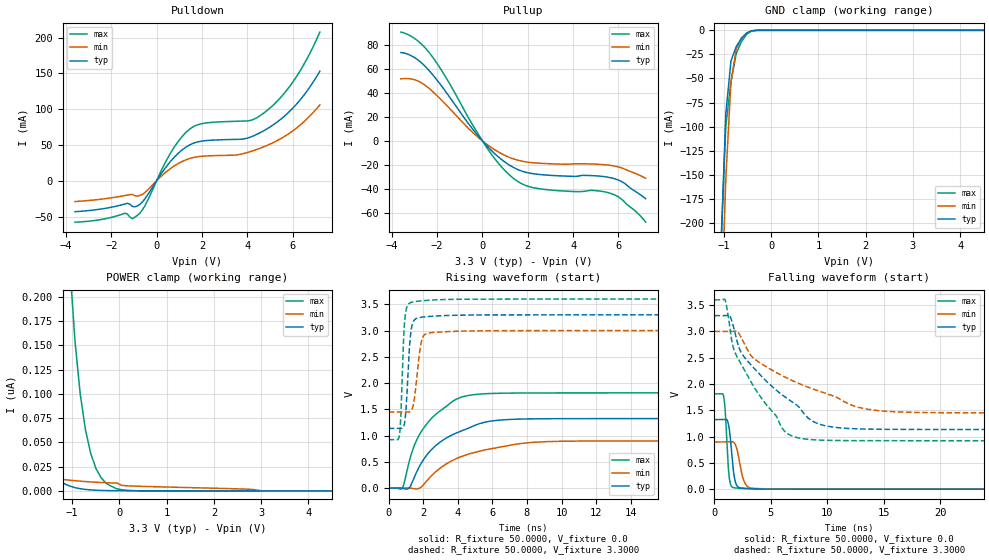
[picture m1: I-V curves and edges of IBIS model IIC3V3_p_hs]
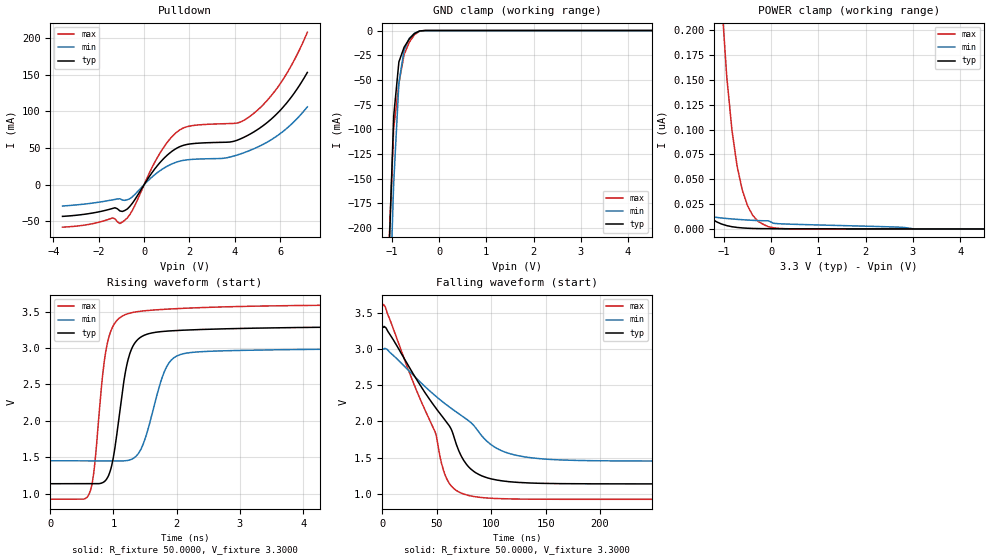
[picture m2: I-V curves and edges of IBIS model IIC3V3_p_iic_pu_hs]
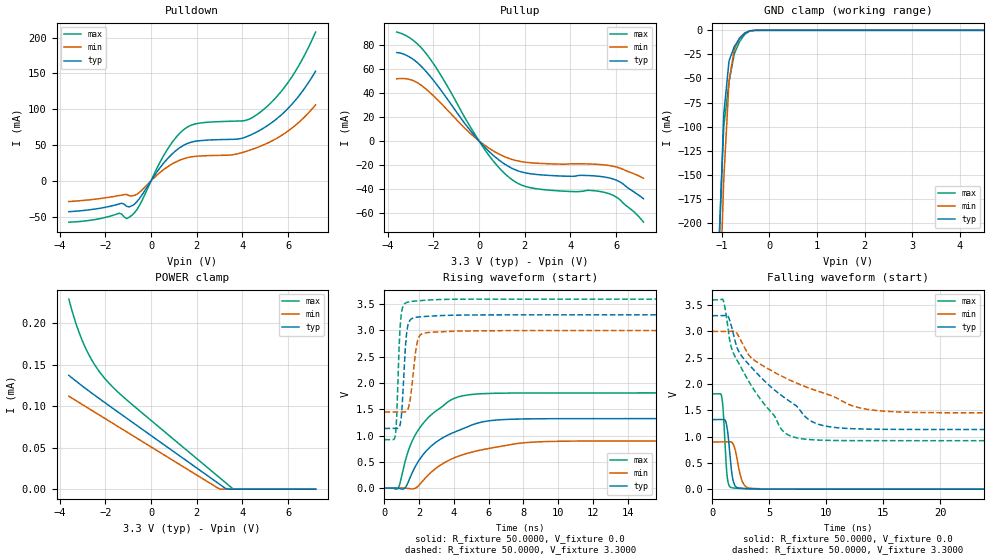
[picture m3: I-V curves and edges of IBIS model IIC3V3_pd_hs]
| IBIS file qfn48_3p3v.ibs generated by Viper version: 2020.12.17
[IBIS Ver]   5.0
[Comment Char]   |_char
[File Name]   qfn48_3p3v.ibs
[File Rev]   1.3
[Date]   Thu Dec 17 17:48:23 2020
[Source]   NXP Viper 2020.12.17
[Notes]
[Disclaimer] IMPORTANT NOTICE
  This information is provided on an AS IS basis and without warranty.
  IN NO EVENT SHALL NXP BE LIABLE FOR INCIDENTAL OR CONSEQUENTIAL
  DAMAGES ARISING FROM USE OF THIS INFORMATION. THIS DISCLAIMER OF
  WARRANTY EXTENDS TO THE USER OF THE INFORMATION, AND TO THEIR CUSTOMERS
  OR USERS OF PRODUCTS  AND IS IN LIEU OF ALL WARRANTIES WHETHER EXPRESS,
  IMPLIED, OR STATUTORY, INCLUDING IMPLIED WARRANTIES OF MERCHANTABILITY
  OR FITNESS FOR PARTICULAR PURPOSE.
  NXP does not represent or warrant that the information furnished
  hereunder is free of infringement of any third party patents,
  copyrights, trade secrets, or other intellectual property rights.
  NXP does not represent or warrant that the information is free of
  defect, or that it meets any particular standard, requirements or need
  of the user of the infomation or their customers.
  NXP reserves the right to change the information in this file
  without notice.
   http://www.nxp.com
[Copyright]   (C) Copyright NXP 2004 - 2020, All Rights Reserved.
|   qfn48
[Component]   qfn48
[Manufacturer]   NXP
[Package]
| variable   typ   min   max
R_pkg   0.17546   0.085233   0.21913
L_pkg   1.979e-9   1.305e-9   2.456e-9
C_pkg   2.005e-13   1.705e-13   3.136e-13
[Pin] signal_name   model_name   R_pin   L_pin   C_pin
1   OPAMP2_INN   NC   0.19686   2.31e-9   1.975e-13
2   P0_1   gpio   0.19885   2.125e-9  1.995e-13
3   P1_0   gpio   0.18462   1.924e-9  1.916e-13
4   P0_11   gpio   0.16868   1.868e-9  1.705e-13
5   VDDIO_1   POWER   NA   NA   NA
6   VDDA   POWER   NA   NA   NA
7   VREF_OUT   NC   0.085233  1.305e-9  2.26e-13
8   VREFP   NC   0.088717  1.309e-9  2.417e-13
9   VREFN   GND   NA   NA   NA
10   P0_16   gpio   0.17435   1.987e-9  1.764e-13
11   P0_10   gpio   0.18496   2.194e-9  1.962e-13
12   P0_15   gpio   0.20527   2.456e-9  2.081e-13
13   P0_8   gpio   0.19119   2.293e-9  1.955e-13
14   OPAMP0_INN   NC   0.1741   2.073e-9  2.101e-13
15   P0_27   gpio   0.16311   1.909e-9  1.814e-13
16   OPAMP1_INN   NC   0.16129   1.801e-9  1.909e-13
17   RESETN   gpio   0.16527   1.717e-9  1.895e-13
18   VDD_CORE   POWER   NA   NA   NA
19   P0_17   gpio   0.16074   1.801e-9  1.861e-13
20   P0_7   gpio   0.1631   1.762e-9  1.925e-13
21   VDDIO_1   POWER   NA   NA   NA
22   VSS_MAIN   GND   NA   NA   NA
23   LX   NC   0.10755   1.361e-9  3.136e-13
24   VDD_MAIN_PWR   NC   NA   NA   NA
25   VBAT   NC   0.21039   2.199e-9  2.126e-13
26   P0_0   gpio   0.19752   2.015e-9  2.122e-13
27   P0_9   gpio   0.17432   1.951e-9  1.886e-13
28   P0_18   gpio   0.16396   1.852e-9  1.719e-13
29   P1_1   gpio   0.1654   1.786e-9  1.75e-13
30   P0_26   gpio   0.16144   1.856e-9  1.764e-13
31   P1_2   gpio   0.16991   1.948e-9  1.848e-13
32   P1_3   gpio   0.18887   2.054e-9  1.928e-13
33   P0_24   gpio   0.17001   1.885e-9  1.791e-13
34   P0_13   iic   0.18016   2.084e-9  1.944e-13
35   P0_14   iic   0.19867   2.298e-9  2.017e-13
36   P0_20   gpio   0.21913   2.324e-9  2.127e-13
37   P0_21   gpio   0.20869   2.216e-9  2.193e-13
38   P0_2   gpio   0.21473   2.265e-9  2.308e-13
39   P0_19   gpio   0.18997   2.14e-9   2.172e-13
40   P0_3   gpio   0.17488   1.926e-9  2.022e-13
41   VDDIO_2   POWER   NA   NA   NA
42   P0_4   gpio   0.16342   1.796e-9  1.814e-13
43   P0_6   gpio   0.16772   1.736e-9  1.992e-13
44   P0_5   gpio   0.16504   1.891e-9  1.879e-13
45   P0_29   gpio   0.16929   1.996e-9  1.98e-13
46   P1_11   gpio   0.18558   2.171e-9  1.964e-13
47   P0_30   gpio   0.20664   2.318e-9  2.205e-13
48   P2_1   gpio   0.1989   2.278e-9  1.972e-13
49   VSS   GND   NA   NA   NA
[Pin Mapping]   pulldown_ref   pullup_ref
1   NC   NC
2   VSS   VDDA
3   VSS   VDDA
4   VSS   VDDA
5   NC   VDDIO_1
6   NC   VDDA
7   NC   NC
8   NC   NC
9   VREFN   NC
10   VSS   VDDA
11   VSS   VDDA
12   VSS   VDDA
13   VSS   VDDA
14   NC   NC
15   VSS   VDDA
16   NC   NC
17   VSS   VDDIO_1
18   NC   VDD_CORE
19   VSS   VDDIO_1
20   VSS   VDDIO_1
21   NC   VDDIO_1
22   VSS_MAIN   NC
23   NC   NC
24   NC   NC
25   NC   NC
26   VSS   VDDIO_2
27   VSS   VDDIO_2
28   VSS   VDDIO_2
29   VSS   VDDIO_2
30   VSS   VDDIO_2
31   VSS   VDDIO_2
32   VSS   VDDIO_2
33   VSS   VDDIO_2
34   VSS   VDDIO_2
35   VSS   VDDIO_2
36   VSS   VDDIO_2
37   VSS   VDDIO_2
38   VSS   VDDIO_2
39   VSS   VDDIO_2
40   VSS   VDDIO_2
41   NC   VDDIO_2
42   VSS   VDDIO_2
43   VSS   VDDIO_2
44   VSS   VDDIO_2
45   VSS   VDDIO_2
46   VSS   VDDIO_2
47   VSS   VDDIO_2
48   VSS   VDDA
49   VSS   NC
|*   Model Selector   *
[Model Selector] gpio
MFIO3V3_pd_hs   EPUN=1 EPD=1 EHS=1
MFIO3V3_pd_ls   EPUN=1 EPD=1 EHS=0
MFIO3V3_pu_hs   EPUN=0 EPD=0 EHS=1
MFIO3V3_pu_ls   EPUN=0 EPD=0 EHS=0
MFIO3V3_p_hs   EPUN=1 EPD=0 EHS=1
MFIO3V3_p_ls   EPUN=1 EPD=0 EHS=0
MFIO3V3_r_hs   EPUN=0 EPD=1 EHS=1
MFIO3V3_r_ls   EPUN=0 EPD=1 EHS=0
[Model Selector] iic
IIC3V3_pd_hs   EGP=1 EPUN=1 EPD=1 EHS=1
IIC3V3_pd_ls   EGP=1 EPUN=1 EPD=1 EHS=0
IIC3V3_p_hs   EGP=1 EPUN=1 EPD=0 EHS=1
IIC3V3_p_ls   EGP=1 EPUN=1 EPD=0 EHS=0
IIC3V3_pu_hs   EGP=1 EPUN=0 EPD=0 EHS=1
IIC3V3_pu_ls   EGP=1 EPUN=0 EPD=0 EHS=0
IIC3V3_r_hs   EGP=1 EPUN=0 EPD=1 EHS=1
IIC3V3_r_ls   EGP=1 EPUN=0 EPD=1 EHS=0
IIC3V3_pd_iic_hs   EGP=0 ECS=0 EPUN=1 EPD=1
IIC3V3_p_iic_hs   EGP=0 ECS=0 EPUN=1 EPD=0
IIC3V3_pu_iic_hs   EGP=0 ECS=0 EPUN=0 EPD=0
IIC3V3_r_iic_hs   EGP=0 ECS=0 EPUN=0 EPD=1
IIC3V3_pd_iic_pu_hs   EGP=0 ECS=1 EPUN=1 EPD=1 SSEL=1
IIC3V3_p_iic_pu_hs   EGP=0 ECS=1 EPUN=1 EPD=0 SSEL=1
IIC3V3_pu_iic_pu_hs   EGP=0 ECS=1 EPUN=0 EPD=0 SSEL=1
IIC3V3_r_iic_pu_hs   EGP=0 ECS=1 EPUN=0 EPD=1 SSEL=1
| End [Component] qfn48
| Models and submodels in the file (24): IIC3V3_p_hs (I/O), IIC3V3_p_iic_hs (I/O_open_drain), IIC3V3_p_iic_pu_hs (I/O_open_drain), IIC3V3_p_ls (I/O), IIC3V3_pd_hs (I/O), IIC3V3_pd_iic_hs (I/O_open_drain), IIC3V3_pd_iic_pu_hs (I/O_open_drain), IIC3V3_pd_ls (I/O), IIC3V3_pu_hs (I/O), IIC3V3_pu_iic_hs (I/O_open_drain), IIC3V3_pu_iic_pu_hs (I/O_open_drain), IIC3V3_pu_ls (I/O), IIC3V3_r_hs (I/O), IIC3V3_r_iic_hs (I/O_open_drain), IIC3V3_r_iic_pu_hs (I/O_open_drain), IIC3V3_r_ls (I/O), MFIO3V3_p_hs (I/O), MFIO3V3_p_ls (I/O), MFIO3V3_pd_hs (I/O), MFIO3V3_pd_ls (I/O), MFIO3V3_pu_hs (I/O), MFIO3V3_pu_ls (I/O), MFIO3V3_r_hs (I/O), MFIO3V3_r_ls (I/O)
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[Model] IIC3V3_p_hs
|   Model IIC3V3_p_hs
| This model was characterised for following simulation conditions:
| External (pad) voltage:
|   - Typ: 3.3V,   - Min: 3.0V,   - Max: 3.6V
| Library cells for typ/min/max conditions are connected as defined below:
|  IO - External Pad
|  A - Core Input
|  EN - Output Buffer Enable
|  BOOST - vdde
|  EGP - vdd
|  EHS - vdd
|  ENZI - vdd
|  EPD - gnd
|  EPUN - vdd
|  ZI - NC
|  ZIF - NC
|  gnd - gnd
|  gnde - gnde
|  vdd - vdd
|  vdde - vdde
| All other pins connected to ground
Model_type I/O
Polarity   Non-Inverting
Enable   Active-Low
Vinl =   0.9900V
Vinh =   2.3100V
Vmeas =  1.6500V
Cref =   0.0F
Rref =   1.0000k
Vref =   0.0V
C_comp   3.6227pF   3.4779pF   3.7656pF
|C_comp_pullup   0.9287pF   0.9115pF   0.9356pF
|C_comp_pulldown   2.3426pF   2.4945pF   2.1982pF
[Model Spec]
| variable   typ   min   max
Vinh   0.9900V   0.9000V   1.0800V
Vinl   2.3100V   2.1000V   2.5200V
Vmeas   1.6500V   1.5000V   1.8000V
[Temperature Range]   25.0000   0.1250k   -40.0000
[Voltage Range]   3.3000V   3.0000V   3.6000V
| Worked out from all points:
|   slope of the pulldown table from 0 to 0.495 V, typ, clamps not added: 22 ohm
|   slope of the pullup table from 0 to 0.495 V, typ, clamps not added: 50.2 ohm
|   GND clamp passes 1 mA (typ) near -0.43 V on its own axis
|   rising waveform, R_fixture 50.0000, V_fixture 0.0: 20-80 % time 2.42ns typ, 3.15ns min, 1.81ns max; typ from 0 V to 1.32 V
|   rising waveform, R_fixture 50.0000, V_fixture 3.3000: 20-80 % time 230ps typ, 322ps min, 186ps max; typ from 1.14 V to 3.3 V
|   falling waveform, R_fixture 50.0000, V_fixture 0.0: 20-80 % time 371ps typ, 535ps min, 282ps max; typ from 1.32 V to 0 V
|   falling waveform, R_fixture 50.0000, V_fixture 3.3000: 20-80 % time 5.52ns typ, 7.85ns min, 3.84ns max; typ from 3.3 V to 1.14 V
[Pulldown]
|Voltage   I(typ)   I(min)   I(max)
-3.6V     -43.22mA   -29.09mA   -57.9mA
-1.29V    -31.46mA   -20.15mA   -46.47mA
-1.07V    -35.79mA   -19.19mA   -52.9mA
-850mV    -35.14mA   -21.36mA   -48.43mA
-520mV    -25.35mA   -16.52mA   -35.11mA
580mV     25.81mA    16.3mA     36.8mA
1.24V     45.79mA    28.53mA    65.82mA
1.9V      54.89mA    33.9mA     79.08mA
4.1V      60.56mA    40.39mA    84.05mA
4.76V     70.46mA    47.89mA    95.34mA
6.08V     103.9mA    71.43mA    141.2mA
7.2V      153mA      106.1mA    207.7mA
[Pullup]
|Voltage   I(typ)   I(min)   I(max)
-3.6V     73.7mA     51.87mA    90.79mA
-2.92V    68.56mA    50.58mA    84.45mA
-2.26V    56.64mA    42.24mA    71.49mA
-1.6V     40.55mA    30.05mA    52.55mA
160mV     -3.402mA   -2.371mA   -4.704mA
820mV     -15.2mA    -10.46mA   -21.22mA
1.37V     -22.16mA   -15.02mA   -31.28mA
1.81V     -25.65mA   -17.18mA   -36.45mA
2.47V     -27.92mA   -18.56mA   -39.79mA
5.66V     -30.76mA   -20.47mA   -43.83mA
6.1V      -33.55mA   -22.29mA   -48.04mA
7.2V      -48.27mA   -31.2mA    -67.82mA
[GND_clamp]
|Voltage   I(typ)   I(min)   I(max)
-3.6V     -5.602A    -5.487A    -5.717A
-1.07V    -242mA     -316.8mA   -230.5mA
-960mV    -86.75mA   -154.7mA   -99.48mA
-850mV    -31.81mA   -53.08mA   -53.5mA
-740mV    -16.96mA   -19.87mA   -24.43mA
-630mV    -8.589mA   -7.919mA   -11.88mA
-520mV    -2.996mA   -2.727mA   -4.187mA
-410mV    -432.5uA   -495.8uA   -580.8uA
7.2V      0A         0A         0A
[POWER_clamp]
|Voltage   I(typ)   I(min)   I(max)
-3.6V     2.12uA     118.8nA    63.41uA
-3.03V    844.5nA    61.84nA    27.62uA
-2.37V    225.8nA    29.91nA    8.403uA
-2.04V    102.5nA    21.72nA    4.105uA
-1.82V    57.11nA    17.98nA    2.406uA
-1.49V    21.61nA    14.11nA    975.4nA
-1.05V    4.967nA    11.05nA    231.3nA
-830mV    2.261nA    10.06nA    99.54nA
-720mV    1.525nA    9.658nA    63.01nA
-500mV    718.9pA    8.985nA    23.37nA
-170mV    294.4pA    8.237nA    4.755nA
7.2V      0A         0A         0A
[Ramp]
| variable   typ   min   max
dV/dt_r  0.7941/2.4211n   0.5390/3.1525n   1.0875/1.8120n
dV/dt_f  1.2989/5.5187n   0.9297/7.8507n   1.6070/3.8381n
R_load = 50.0000
[Rising Waveform]
R_fixture= 50.0000
V_fixture= 0.0
V_fixture_min= 0.0
V_fixture_max= 0.0
|time   V(typ)   V(min)   V(max)
0s        2.243nV    52.63nV    27.54nV
783.4ps   -2.546mV   48.23uV    -3.663mV
1.2ns     6.371mV    -1.183mV   516.9mV
1.762ns   400.2mV    -5.572mV   1.005V
2.604ns   772.3mV    274.8mV    1.368V
3.633ns   1.006V     515.9mV    1.636V
5.446ns   1.245V     716.8mV    1.794V
7.589ns   1.314V     845.6mV    1.81V
17.45ns   1.323V     898mV      1.812V
1us       1.323V     898.3mV    1.813V
[Rising Waveform]
R_fixture= 50.0000
V_fixture= 3.3000
V_fixture_min= 3.0000
V_fixture_max= 3.6000
|time   V(typ)   V(min)   V(max)
0s        1.135V     1.45V      921.7mV
627.3ps   1.135V     1.45V      1.012V
700.7ps   1.134V     1.451V     1.326V
903.6ps   1.208V     1.45V      3.068V
1.101ns   2.057V     1.448V     3.484V
1.223ns   2.763V     1.454V     3.525V
1.356ns   3.105V     1.506V     3.542V
2.023ns   3.26V      2.9V       3.57V
4.301ns   3.294V     2.99V      3.597V
1us       3.3V       3V         3.6V
[Falling Waveform]
R_fixture= 50.0000
V_fixture= 0.0
V_fixture_min= 0.0
V_fixture_max= 0.0
|time   V(typ)   V(min)   V(max)
0s        1.323V     898.3mV    1.813V
822ps     1.323V     898.3mV    1.758V
972.4ps   1.326V     898.3mV    1.431V
1.252ns   1.222V     898.1mV    350.6mV
1.476ns   816.9mV    900.3mV    64.93mV
1.726ns   277.3mV    889.4mV    27.64mV
2.019ns   57.27mV    737.3mV    19.74mV
2.754ns   14.85mV    95.71mV    10.98mV
4.273ns   3.379mV    7.479mV    1.748mV
1us       13.95nV    73.04nV    34.74nV
[Falling Waveform]
R_fixture= 50.0000
V_fixture= 3.3000
V_fixture_min= 3.0000
V_fixture_max= 3.6000
|time   V(typ)   V(min)   V(max)
0s        3.3V       3V         3.6V
933.7ps   3.299V     3V         3.603V
1.389ns   3.287V     2.999V     3.037V
1.891ns   2.917V     3.01V      2.567V
2.697ns   2.498V     2.747V     2.246V
6.123ns   1.774V     2.146V     1.125V
10.95ns   1.17V      1.732V     925.1mV
14.46ns   1.14V      1.495V     922mV
24.74ns   1.135V     1.451V     921.7mV
1us       1.135V     1.45V      921.7mV
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[Model] IIC3V3_p_iic_pu_hs
|   Model IIC3V3_p_iic_pu_hs
| This model was characterised for following simulation conditions:
| External (pad) voltage:
|   - Typ: 3.3V,   - Min: 3.0V,   - Max: 3.6V
| Library cells for typ/min/max conditions are connected as defined below:
|  IO - External Pad
|  A - Core Input
|  EN - Output Buffer Enable
|  BOOST - vdde
|  ECS - vdd
|  EGP - gnd
|  ENZI - vdd
|  EPD - gnd
|  EPUN - vdd
|  SSEL - vdd
|  ZI - NC
|  ZIF - NC
|  gnd - gnd
|  gnde - gnde
|  vdd - vdd
|  vdde - vdde
| All other pins connected to ground
Model_type I/O_open_drain
Polarity   Non-Inverting
Enable   Active-Low
Vinl =   0.9900V
Vinh =   2.3100V
Vmeas =  1.6500V
Cref =   0.0F
Rref =   1.0000k
Vref =   3.3000V
C_comp   3.6227pF   3.4779pF   3.7656pF
|C_comp_pullup   0.9287pF   0.9114pF   0.9356pF
|C_comp_pulldown   2.3426pF   2.4946pF   2.1982pF
[Model Spec]
| variable   typ   min   max
Vinh   0.9900V   0.9000V   1.0800V
Vinl   2.3100V   2.1000V   2.5200V
Vmeas   1.6500V   1.5000V   1.8000V
Vref   3.3000V   3.0000V   3.6000V
Cref   0.0F   0.0F   0.0F
Rref   1.0000k   1.0000k   1.0000k
[Temperature Range]   25.0000   0.1250k   -40.0000
[Voltage Range]   3.3000V   3.0000V   3.6000V
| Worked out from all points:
|   slope of the pulldown table from 0 to 0.495 V, typ, clamps not added: 22 ohm
|   GND clamp passes 1 mA (typ) near -0.43 V on its own axis
|   rising waveform, R_fixture 50.0000, V_fixture 3.3000: 20-80 % time 227ps typ, 309ps min, 192ps max; typ from 1.14 V to 3.3 V
|   falling waveform, R_fixture 50.0000, V_fixture 3.3000: 20-80 % time 50.8ns typ, 68.7ns min, 38.5ns max; typ from 3.3 V to 1.14 V
[Pulldown]
|Voltage   I(typ)   I(min)   I(max)
-3.6V     -43.22mA   -29.09mA   -57.9mA
-1.29V    -31.46mA   -20.15mA   -46.47mA
-1.07V    -35.79mA   -19.19mA   -52.9mA
-850mV    -35.14mA   -21.36mA   -48.43mA
-520mV    -25.35mA   -16.52mA   -35.11mA
580mV     25.81mA    16.3mA     36.8mA
1.24V     45.79mA    28.53mA    65.82mA
1.9V      54.89mA    33.9mA     79.08mA
4.1V      60.56mA    40.39mA    84.05mA
4.76V     70.46mA    47.89mA    95.34mA
6.08V     103.9mA    71.43mA    141.2mA
7.2V      153mA      106.1mA    207.7mA
[GND_clamp]
|Voltage   I(typ)   I(min)   I(max)
-3.6V     -5.602A    -5.487A    -5.717A
-1.07V    -242mA     -316.8mA   -230.5mA
-960mV    -86.75mA   -154.7mA   -99.48mA
-850mV    -31.81mA   -53.08mA   -53.5mA
-740mV    -16.96mA   -19.87mA   -24.43mA
-630mV    -8.589mA   -7.919mA   -11.88mA
-520mV    -2.996mA   -2.727mA   -4.187mA
-410mV    -432.5uA   -495.8uA   -580.8uA
7.2V      0A         0A         0A
[POWER_clamp]
|Voltage   I(typ)   I(min)   I(max)
-3.6V     2.12uA     118.8nA    63.41uA
-3.03V    844.5nA    61.84nA    27.62uA
-2.37V    225.8nA    29.91nA    8.403uA
-2.04V    102.5nA    21.72nA    4.105uA
-1.82V    57.11nA    17.98nA    2.406uA
-1.49V    21.61nA    14.11nA    975.4nA
-1.05V    4.967nA    11.05nA    231.3nA
-830mV    2.261nA    10.06nA    99.54nA
-720mV    1.525nA    9.658nA    63.01nA
-500mV    718.9pA    8.985nA    23.37nA
-170mV    294.4pA    8.237nA    4.755nA
7.2V      0A         0A         0A
[Ramp]
| variable   typ   min   max
dV/dt_r  1.2989/0.2271n   0.9297/0.3090n   1.6070/0.1925n
dV/dt_f  1.2989/50.7796n   0.9297/68.6526n   1.6070/38.5019n
R_load = 50.0000
[Rising Waveform]
R_fixture= 50.0000
V_fixture= 3.3000
V_fixture_min= 3.0000
V_fixture_max= 3.6000
|time   V(typ)   V(min)   V(max)
0s        1.135V     1.45V      921.7mV
623.4ps   1.135V     1.45V      1.013V
886ps     1.193V     1.45V      2.995V
994ps     1.479V     1.45V      3.305V
1.153ns   2.48V      1.449V     3.448V
1.388ns   3.122V     1.544V     3.503V
1.807ns   3.231V     2.682V     3.534V
2.03ns    3.244V     2.903V     3.544V
5.603ns   3.294V     2.992V     3.595V
1us       3.3V       3V         3.6V
[Falling Waveform]
R_fixture= 50.0000
V_fixture= 3.3000
V_fixture_min= 3.0000
V_fixture_max= 3.6000
|time   V(typ)   V(min)   V(max)
0s        3.3V       3V         3.6V
2.46ns    3.303V     3.01V      3.593V
48.38ns   2.199V     2.358V     1.857V
54.58ns   2.076V     2.28V      1.407V
59.71ns   1.976V     2.22V      1.188V
72.76ns   1.512V     2.08V      1.006V
83.18ns   1.317V     1.957V     962.6mV
112.4ns   1.172V     1.577V     928.9mV
163.4ns   1.139V     1.467V     922.1mV
1us       1.135V     1.45V      921.7mV
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[Model] IIC3V3_pd_hs
|   Model IIC3V3_pd_hs
| This model was characterised for following simulation conditions:
| External (pad) voltage:
|   - Typ: 3.3V,   - Min: 3.0V,   - Max: 3.6V
| Library cells for typ/min/max conditions are connected as defined below:
|  IO - External Pad
|  A - Core Input
|  EN - Output Buffer Enable
|  BOOST - vdde
|  EGP - vdd
|  EHS - vdd
|  ENZI - vdd
|  EPD - vdd
|  EPUN - vdd
|  ZI - NC
|  ZIF - NC
|  gnd - gnd
|  gnde - gnde
|  vdd - vdd
|  vdde - vdde
| All other pins connected to ground
Model_type I/O
Polarity   Non-Inverting
Enable   Active-Low
Vinl =   0.9900V
Vinh =   2.3100V
Vmeas =  1.6500V
Cref =   0.0F
Rref =   1.0000k
Vref =   0.0V
C_comp   3.5907pF   3.4406pF   3.7387pF
|C_comp_pullup   0.9138pF   0.9000pF   0.9174pF
|C_comp_pulldown   2.3267pF   2.4802pF   2.1806pF
[Model Spec]
| variable   typ   min   max
Vinh   0.9900V   0.9000V   1.0800V
Vinl   2.3100V   2.1000V   2.5200V
Vmeas   1.6500V   1.5000V   1.8000V
[Temperature Range]   25.0000   0.1250k   -40.0000
[Voltage Range]   3.3000V   3.0000V   3.6000V
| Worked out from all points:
|   slope of the pulldown table from 0 to 0.495 V, typ, clamps not added: 22 ohm
|   slope of the pullup table from 0 to 0.495 V, typ, clamps not added: 50.2 ohm
|   GND clamp passes 1 mA (typ) near -0.43 V on its own axis
|   rising waveform, R_fixture 50.0000, V_fixture 0.0: 20-80 % time 2.41ns typ, 3.15ns min, 1.81ns max; typ from 0 V to 1.32 V
|   rising waveform, R_fixture 50.0000, V_fixture 3.3000: 20-80 % time 230ps typ, 322ps min, 186ps max; typ from 1.14 V to 3.3 V
|   falling waveform, R_fixture 50.0000, V_fixture 0.0: 20-80 % time 371ps typ, 533ps min, 281ps max; typ from 1.32 V to 0 V
|   falling waveform, R_fixture 50.0000, V_fixture 3.3000: 20-80 % time 5.51ns typ, 7.83ns min, 3.82ns max; typ from 3.3 V to 1.14 V
[Pulldown]
|Voltage   I(typ)   I(min)   I(max)
-3.6V     -43.22mA   -29.09mA   -57.9mA
-1.29V    -31.46mA   -20.15mA   -46.47mA
-1.07V    -35.79mA   -19.19mA   -52.9mA
-850mV    -35.14mA   -21.36mA   -48.43mA
-520mV    -25.35mA   -16.52mA   -35.11mA
580mV     25.81mA    16.3mA     36.8mA
1.24V     45.79mA    28.53mA    65.82mA
1.9V      54.89mA    33.9mA     79.08mA
4.1V      60.55mA    40.38mA    84.05mA
4.76V     70.44mA    47.87mA    95.32mA
6.08V     103.9mA    71.39mA    141.2mA
7.2V      152.9mA    106mA      207.6mA
[Pullup]
|Voltage   I(typ)   I(min)   I(max)
-3.6V     73.65mA    51.83mA    90.73mA
-2.92V    68.52mA    50.55mA    84.41mA
-2.26V    56.61mA    42.22mA    71.46mA
-1.6V     40.53mA    30.04mA    52.53mA
160mV     -3.403mA   -2.371mA   -4.704mA
820mV     -15.2mA    -10.46mA   -21.22mA
1.37V     -22.16mA   -15.02mA   -31.28mA
1.81V     -25.65mA   -17.18mA   -36.45mA
2.47V     -27.92mA   -18.56mA   -39.79mA
5.66V     -30.76mA   -20.47mA   -43.83mA
6.1V      -33.55mA   -22.29mA   -48.04mA
7.2V      -48.27mA   -31.2mA    -67.82mA
[GND_clamp]
|Voltage   I(typ)   I(min)   I(max)
-3.6V     -5.602A    -5.487A    -5.717A
-1.07V    -242mA     -316.8mA   -230.5mA
-960mV    -86.76mA   -154.7mA   -99.49mA
-850mV    -31.82mA   -53.09mA   -53.51mA
-740mV    -16.97mA   -19.87mA   -24.44mA
-630mV    -8.597mA   -7.926mA   -11.89mA
-520mV    -3.004mA   -2.733mA   -4.196mA
-410mV    -439.7uA   -501.8uA   -589.4uA
7.2V      0A         0A         0A
[POWER_clamp]
|Voltage   I(typ)   I(min)   I(max)
-3.6V     137uA      111.9uA    228.9uA
-3.47V    134.1uA    109.7uA    215.6uA
-3.25V    129.3uA    106uA      196.2uA
-2.92V    122.3uA    100.4uA    172.9uA
-2.48V    113.3uA    92.88uA    150.2uA
-2.04V    104.5uA    85.42uA    133.7uA
-1.16V    87.2uA     70.51uA    109.7uA
2.91V     7.626uA    1.527uA    15.86uA
3.02V     5.475uA    0A         13.33uA
3.24V     1.173uA    0A         8.273uA
3.57V     0A         0A         687.1nA
7.2V      0A         0A         0A
[Ramp]
| variable   typ   min   max
dV/dt_r  0.7935/2.4144n   0.5386/3.1478n   1.0867/1.8089n
dV/dt_f  1.2983/5.5124n   0.9293/7.8350n   1.6062/3.8243n
R_load = 50.0000
[Rising Waveform]
R_fixture= 50.0000
V_fixture= 0.0
V_fixture_min= 0.0
V_fixture_max= 0.0
|time   V(typ)   V(min)   V(max)
0s        2.145nV    50.58nV    26.14nV
784.7ps   -2.611mV   49.1uV     -3.137mV
1.202ns   7.028mV    -1.221mV   519mV
1.771ns   405.7mV    -4.318mV   1.01V
2.618ns   776.7mV    279.1mV    1.373V
3.639ns   1.007V     517.2mV    1.637V
5.503ns   1.249V     720.8mV    1.794V
7.438ns   1.312V     838.3mV    1.809V
17.91ns   1.322V     897.4mV    1.811V
1us       1.322V     897.6mV    1.811V
[Rising Waveform]
R_fixture= 50.0000
V_fixture= 3.3000
V_fixture_min= 3.0000
V_fixture_max= 3.6000
|time   V(typ)   V(min)   V(max)
0s        1.135V     1.45V      921.3mV
628ps     1.134V     1.45V      1.013V
701.4ps   1.133V     1.45V      1.33V
904.8ps   1.209V     1.449V     3.073V
1.102ns   2.066V     1.447V     3.485V
1.223ns   2.761V     1.453V     3.525V
1.356ns   3.104V     1.505V     3.541V
2.025ns   3.259V     2.9V       3.569V
4.329ns   3.293V     2.989V     3.596V
1us       3.299V     2.999V     3.598V
[Falling Waveform]
R_fixture= 50.0000
V_fixture= 0.0
V_fixture_min= 0.0
V_fixture_max= 0.0
|time   V(typ)   V(min)   V(max)
0s        1.322V     897.6mV    1.811V
823ps     1.322V     897.6mV    1.756V
974.3ps   1.325V     897.6mV    1.423V
1.254ns   1.218V     897.5mV    343.4mV
1.479ns   809.6mV    899.6mV    62.93mV
1.72ns    284.1mV    889.7mV    27.16mV
2.013ns   58.28mV    741.7mV    19.25mV
2.763ns   14.33mV    92.17mV    10.48mV
4.222ns   3.365mV    7.6mV      1.686mV
1us       13.83nV    70.96nV    33.33nV
[Falling Waveform]
R_fixture= 50.0000
V_fixture= 3.3000
V_fixture_min= 3.0000
V_fixture_max= 3.6000
|time   V(typ)   V(min)   V(max)
0s        3.299V     2.999V     3.598V
922.2ps   3.298V     2.999V     3.606V
1.378ns   3.29V      2.998V     3.054V
1.853ns   2.949V     3.007V     2.582V
2.668ns   2.504V     2.757V     2.255V
6.08ns    1.779V     2.149V     1.135V
10.78ns   1.173V     1.748V     925.2mV
14.53ns   1.139V     1.493V     921.7mV
23.45ns   1.135V     1.451V     921.4mV
1us       1.135V     1.45V      921.3mV
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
